(* Logix 5000 AddOnInstructionDefinition export QWX43; software revision 18.02; part 2 of 2 *)
(* tags used below, declared in another part *)
   Inp_Release : BOOL;   // 1= Enable communication to QWX43
   SKT_DATA_Client : SKT_DATA_CLIENT;   // This tags holds all the data used by the messages
   SKT_MSG_Client_Create : MESSAGE;   // Create socket
   SKT_MSG_Client_Connect : MESSAGE;   // Connect socket to server.
   SKT_MSG_Client_Read : MESSAGE;   // Message to tell socket to return any data it has recieved
   SKT_MSG_Client_Write : MESSAGE;   // Write socket message
   SKT_MSG_Client_Delete : MESSAGE;   // Delete socket
   Out_SensorData : QWX43_SensorData;   // Received Sensor Data
   Sts_Error : BOOL;   // 1= functionblock is in an error state
   Sts_State : DINT;   // State of the function 0=Wait, 1=Connect, 2=Send, 3=Receive 100=ConfigError, 101=ConnectionError, 102=TelegramError, 103=
   Err_Config : BOOL;   // Error in basic configuration
   Wrk_State : DINT;   // State of the function 0=Wait, 1=Connect, 2=Send, 3=Receive 100=ConfigError, 101=ConnectionError, 102=TelegramError, 103=
   Wrk_Connected : BOOL;   // Socket is connected to the QWX43
   SKT_AOI_Client : SKT_AOI_TCP_CLIENT;   // Socket handling
   Wrk_ReceiveBuffer : STR_480;
   Err_ReceiveDataLenNOK : BOOL;   // The received data lengh did not match
   Err_ReceiveHeaderDataNOK : BOOL;   // At least one of the received header data was incorrect
   Wrk_ReceiveByteOffset : DINT;
   Wrk_ReceiveByteLen : DINT;
   Wrk_ReceiveSwapIndex : DINT;
   Wrk_ReceiveSwapNo : DINT;   // Number of data elements to swap
   Wrk_ReceiveSwapSize : DINT;   // Number of bytes per element to swap
   Wrk_dummyINT_A : INT[100];
   Wrk_dummyINT_A_Size : DINT;
   Err_ReceiveVersionNOK : BOOL;   // The received data version is incorrect
   Err_Connection : BOOL;   // No connection could be established
   Err_ConnectionTimeout : BOOL;   // Timeout after a connection was established
   Err_MSGDeleteAll : BOOL;   // The MSG Delete All had an error
(* QWX43, continued *)

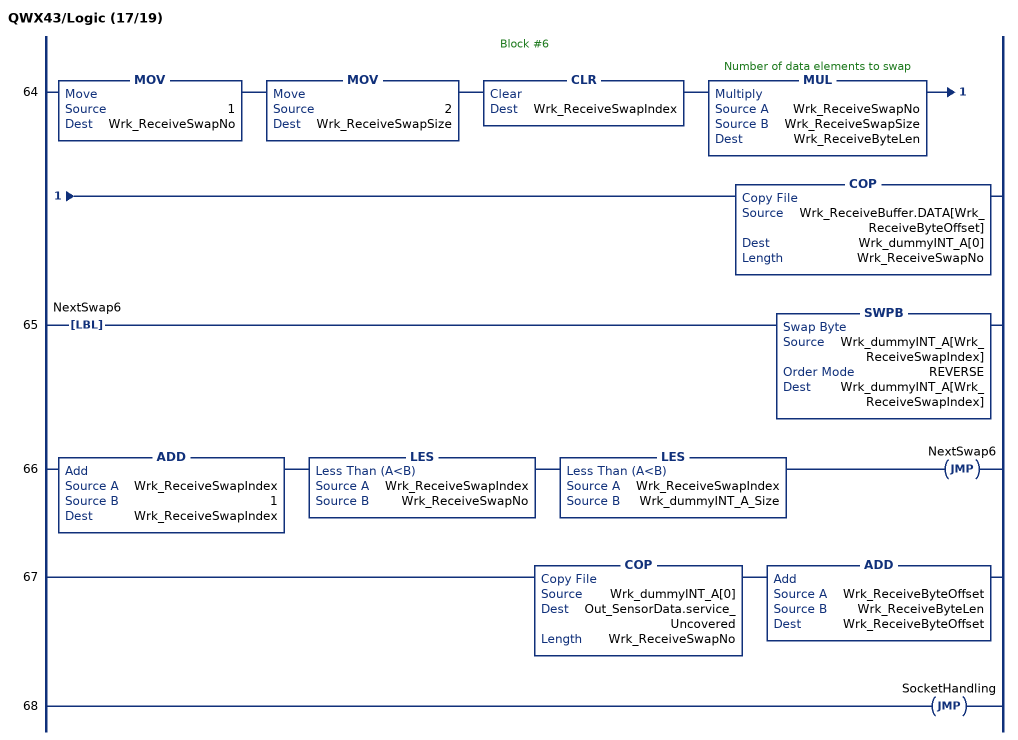
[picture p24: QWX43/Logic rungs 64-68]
   // Block #6
   64: MOV(1,Wrk_ReceiveSwapNo)MOV(2,Wrk_ReceiveSwapSize)CLR(Wrk_ReceiveSwapIndex)MUL(Wrk_ReceiveSwapNo,Wrk_ReceiveSwapSize,Wrk_ReceiveByteLen)COP(Wrk_ReceiveBuffer.DATA[Wrk_ReceiveByteOffset],Wrk_dummyINT_A[0],Wrk_ReceiveSwapNo);
   65: LBL(NextSwap6)SWPB(Wrk_dummyINT_A[Wrk_ReceiveSwapIndex],REVERSE,Wrk_dummyINT_A[Wrk_ReceiveSwapIndex]);
   66: ADD(Wrk_ReceiveSwapIndex,1,Wrk_ReceiveSwapIndex)LES(Wrk_ReceiveSwapIndex,Wrk_ReceiveSwapNo)LES(Wrk_ReceiveSwapIndex,Wrk_dummyINT_A_Size)JMP(NextSwap6);
   67: COP(Wrk_dummyINT_A[0],Out_SensorData.service_Uncovered,Wrk_ReceiveSwapNo)ADD(Wrk_ReceiveByteOffset,Wrk_ReceiveByteLen,Wrk_ReceiveByteOffset);
   68: JMP(SocketHandling);
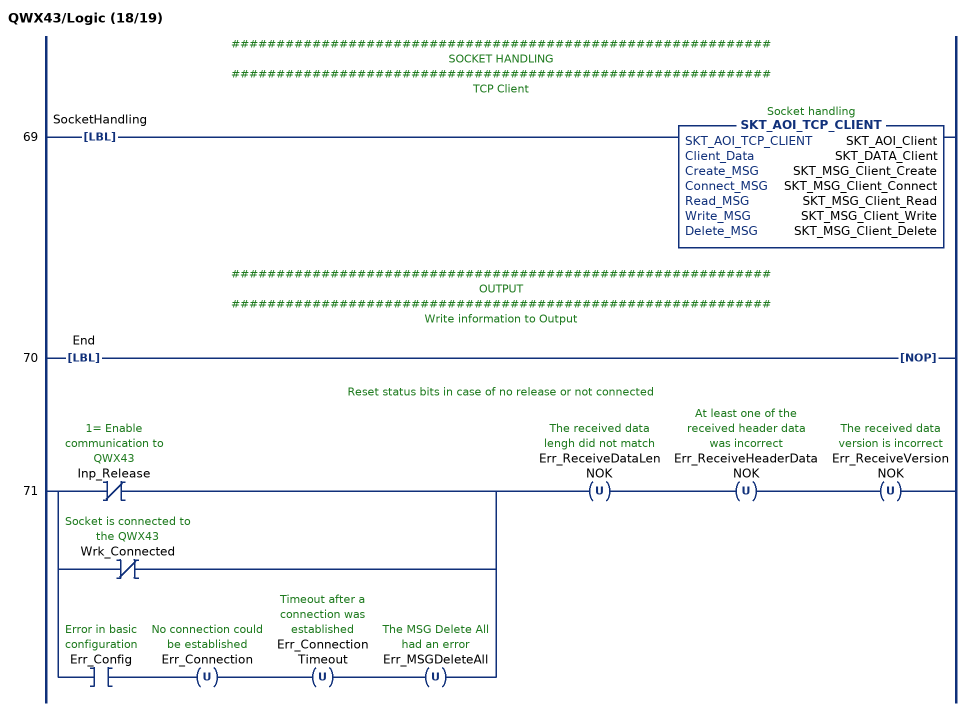
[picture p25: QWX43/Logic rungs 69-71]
   // ############################################################
   // SOCKET HANDLING
   // ############################################################
   // TCP Client
   69: LBL(SocketHandling)SKT_AOI_TCP_CLIENT(SKT_AOI_Client,SKT_DATA_Client,SKT_MSG_Client_Create,SKT_MSG_Client_Connect,SKT_MSG_Client_Read,SKT_MSG_Client_Write,SKT_MSG_Client_Delete);
   // ############################################################
   // OUTPUT
   // ############################################################
   // Write information to Output
   70: LBL(End)NOP();
   // Reset status bits in case of no release or not connected
   71: [[XIO(Inp_Release) ,XIO(Wrk_Connected) ] ,XIC(Err_Config) OTU(Err_Connection) OTU(Err_ConnectionTimeout) OTU(Err_MSGDeleteAll) ]OTU(Err_ReceiveDataLenNOK)OTU(Err_ReceiveHeaderDataNOK)OTU(Err_ReceiveVersionNOK);
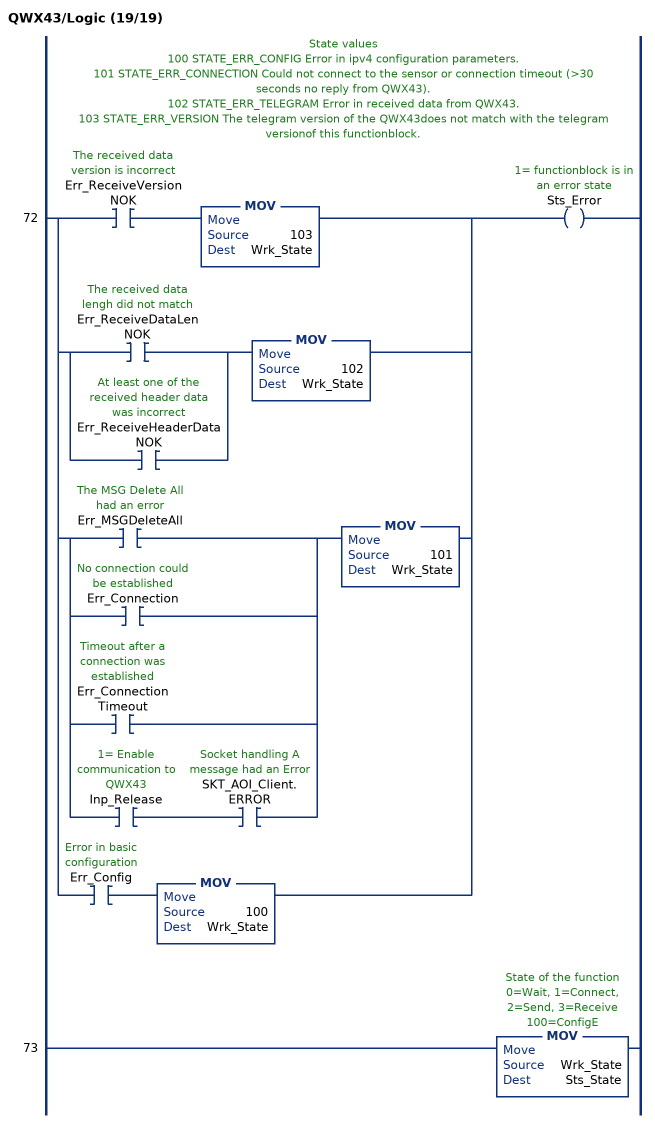
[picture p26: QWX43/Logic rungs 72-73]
   // State values
   // 100 STATE_ERR_CONFIG Error in ipv4 configuration parameters.
   // 101 STATE_ERR_CONNECTION Could not connect to the sensor or connection timeout (>30 seconds no reply from QWX43).
   // 102 STATE_ERR_TELEGRAM Error in received data from QWX43.
   // 103 STATE_ERR_VERSION The telegram version of the QWX43does not match with the telegram versionof this functionblock.
   72: [XIC(Err_ReceiveVersionNOK) MOV(103,Wrk_State) ,[XIC(Err_ReceiveDataLenNOK) ,XIC(Err_ReceiveHeaderDataNOK) ] MOV(102,Wrk_State) ,[XIC(Err_MSGDeleteAll) ,XIC(Err_Connection) ,XIC(Err_ConnectionTimeout) ,XIC(Inp_Release) XIC(SKT_AOI_Client.ERROR) ] MOV(101,Wrk_State) ,XIC(Err_Config) MOV(100,Wrk_State) ]OTE(Sts_Error);
   73: MOV(Wrk_State,Sts_State);
END_ROUTINE
END_ADD_ON_INSTRUCTION
